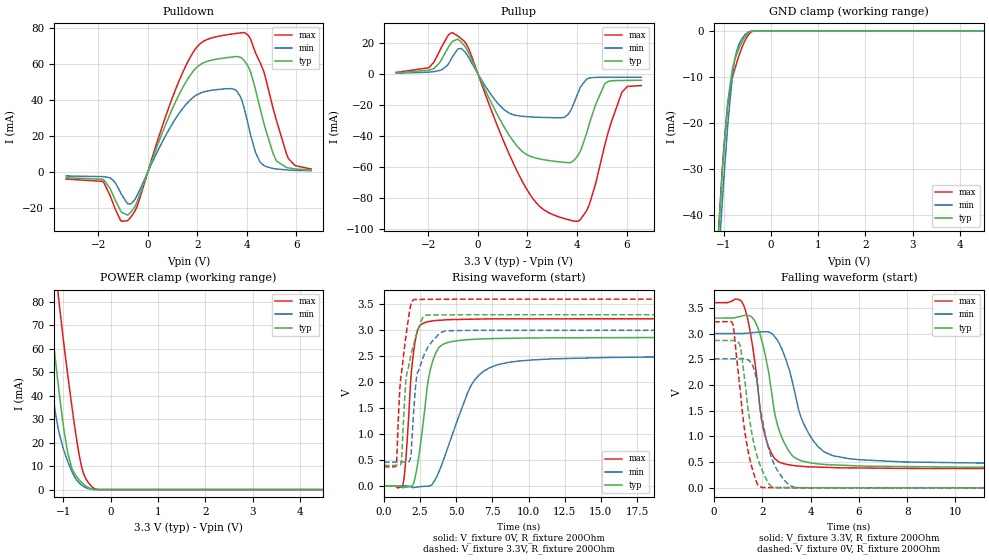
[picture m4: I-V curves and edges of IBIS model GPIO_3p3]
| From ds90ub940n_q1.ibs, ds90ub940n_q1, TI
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|   Model
[Model]   GPIO_3p3
Model_type   I/O
Polarity   Non-Inverting
Enable   Active-Low
Vinl = 0.8
Vinh = 2.0
Vmeas = 1.65
Vref = 0
Cref = 1pF
Rref = 100000
|   typ   min   max
C_comp   1.5999pF   1.5084pF   1.9148pF
[Voltage Range]   3.3   3   3.6
[Temperature Range]   27   105   -40
[Pullup Reference]   3.3   3   3.6
[Pulldown Reference]   -0   0   0
[Power Clamp Reference]   3.3   3   3.6
[GND Clamp Reference]   0   0   0
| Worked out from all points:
|   slope of the pulldown table from 0 to 0.495 V, typ, clamps not added: 26.6 ohm
|   slope of the pullup table from 0 to 0.495 V, typ, clamps not added: 29 ohm
|   GND clamp passes 1 mA (typ) near -0.52 V on its own axis
|   POWER clamp passes 1 mA (typ) near -0.48 V on its own axis
|   falling waveform, V_fixture 3.3V, R_fixture 200Ohm: 20-80 % time 759ps typ, 1.06ns min, 587ps max; typ from 3.3 V to 0.396 V
|   rising waveform, V_fixture 0V, R_fixture 200Ohm: 20-80 % time 842ps typ, 2.07ns min, 504ps max; typ from 0 V to 2.86 V
|   rising waveform, V_fixture 3.3V, R_fixture 200Ohm: 20-80 % time 741ps typ, 779ps min, 598ps max; typ from 0.395 V to 3.3 V
|   falling waveform, V_fixture 0V, R_fixture 200Ohm: 20-80 % time 590ps typ, 660ps min, 516ps max; typ from 2.87 V to 0 V
[Pulldown]
|   Voltage   I(typ)   I(min)   I(max)
-3.3V     -3.164mA   -2.173mA   -3.905mA
-1.835V   -3.993mA   -2.542mA   -5.143mA
-1.112V   -21.25mA   -11.09mA   -26.52mA
-815.1mV  -23.91mA   -17.65mA   -27.01mA
-429mV    -16.44mA   -12.96mA   -18.93mA
1.818V    55.76mA    41.37mA    66.26mA
3.482V    64.03mA    46.04mA    76.84mA
3.877V    62.19mA    36.29mA    77.51mA
4.531V    35.47mA    5.597mA    60.97mA
5.184V    6.455mA    1.721mA    29.19mA
5.679V    2.299mA    1.122mA    7.433mA
6.6V      1.091mA    735.9uA    1.663mA
[GND Clamp]
|   Voltage   I(typ)   I(min)   I(max)
-3.3V     -490.9mA   -454.2mA   -525.1mA
-1.122V   -47.07mA   -52.59mA   -46.26mA
-1.033V   -32.05mA   -38.23mA   -31.12mA
-993.3mV  -26.03mA   -32.18mA   -25.39mA
-914.1mV  -15.95mA   -21mA      -16.38mA
-815.1mV  -8.436mA   -9.999mA   -10.35mA
-755.7mV  -6.108mA   -5.891mA   -8.109mA
-686.4mV  -4.119mA   -3.295mA   -5.787mA
-577.5mV  -1.834mA   -1.244mA   -2.814mA
-458.7mV  -332.6uA   -204.8uA   -676.2uA
-260.7mV  -1.284uA   -1.62uA    -2.04uA
6.6V      0A         0A         0A
[Pullup]
|   Voltage   I(typ)   I(min)   I(max)
-3.3V     727.6uA    454.7uA    986.5uA
-1.993V   2.271mA    1.124mA    3.904mA
-1.468V   9.315mA    2.642mA    17.31mA
-676.5mV  20.61mA    16.42mA    22.71mA
768.9mV   -25.77mA   -18.3mA    -32.8mA
1.68V     -48.24mA   -27.07mA   -65.82mA
2.511V    -54.85mA   -27.98mA   -85.64mA
3.897V    -55.4mA    -18mA      -94.88mA
4.501V    -32.01mA   -2.633mA   -84.1mA
5.115V    -6.534mA   -2.196mA   -46.4mA
5.818V    -4.217mA   -2.156mA   -11.71mA
6.6V      -4.115mA   -2.126mA   -7.516mA
[POWER Clamp]
|   Voltage   I(typ)   I(min)   I(max)
-3.3V     488.4mA    415.5mA    566.2mA
-1.676V   153.8mA    114.9mA    202.9mA
-1.409V   100.9mA    68.98mA    144.9mA
-1.35V    89.41mA    59.34mA    132.2mA
-1.231V   66.97mA    41.31mA    107.5mA
-1.102V   43.92mA    25.52mA    82.16mA
-973.5mV  23.72mA    15.84mA    59.7mA
-815.1mV  8.895mA    7.566mA    34.94mA
-636.9mV  3.54mA     2.322mA    11.95mA
-508.2mV  1.311mA    677.8uA    4.14mA
-260.7mV  6.871uA    4.277uA    41.53uA
6.6V      0A         0A         0A
[Ramp]
R_load = 200
|   typ   min   max
dV/dt_r   1.71827/8.41806e-10   1.50408/2.06636e-09   1.93592/5.02199e-10
dV/dt_f   1.74251/7.59472e-10   1.52289/1.05507e-09   1.93753/5.8591e-10
[Falling Waveform]
V_fixture = 3.3V
V_fixture_min = 3V
V_fixture_max = 3.6V
R_fixture = 200Ohm
C_fixture = 0F
|   Time   V(typ)   V(min)   V(max)
0s        3.3V       3V         3.6V
1.161ns   3.341V     3.001V     3.609V
1.693ns   3.239V     3.021V     2.43V
1.959ns   2.893V     3.032V     1.352V
2.26ns    2.25V      3.031V     798.1mV
2.611ns   1.252V     2.881V     531.3mV
3.175ns   667.5mV    2.191V     441.9mV
4.176ns   473.8mV    875.1mV    406mV
5.811ns   430.4mV    556.1mV    387.3mV
40ns      395.8mV    461.8mV    370.8mV
[Rising Waveform]
V_fixture = 0V
V_fixture_min = 0V
V_fixture_max = 0V
R_fixture = 200Ohm
C_fixture = 0F
|   Time   V(typ)   V(min)   V(max)
0s        -6.538uV   984.3nV    3.936uV
1.291ns   -31.74mV   17.28uV    2.32mV
1.505ns   -25.18mV   19.97uV    480.4mV
1.863ns   -6.233mV   -16.06mV   2.073V
2.085ns   86.31mV    -29.62mV   2.651V
2.983ns   1.882V     -4.527mV   3.161V
4.041ns   2.725V     442.5mV    3.197V
6.047ns   2.823V     1.949V     3.213V
7.86ns    2.842V     2.337V     3.22V
40ns      2.864V     2.507V     3.227V
[Rising Waveform]
V_fixture = 3.3V
V_fixture_min = 3V
V_fixture_max = 3.6V
R_fixture = 200Ohm
C_fixture = 0F
|   Time   V(typ)   V(min)   V(max)
0s        395.4mV    460.8mV    370.5mV
856.2ps   394.2mV    460.6mV    416.7mV
1.182ns   433mV      460.6mV    2.118V
1.548ns   2.109V     460.5mV    2.943V
1.857ns   2.508V     578.2mV    3.49V
2.085ns   2.76V      1.548V     3.591V
2.272ns   2.928V     2.129V     3.594V
2.811ns   3.275V     2.549V     3.595V
4.327ns   3.296V     2.991V     3.598V
40ns      3.3V       3V         3.6V
[Falling Waveform]
|Gnd
V_fixture = 0V
V_fixture_min = 0V
V_fixture_max = 0V
R_fixture = 200Ohm
C_fixture = 0F
|   Time   V(typ)   V(min)   V(max)
0s        2.865V     2.507V     3.227V
778.2ps   2.865V     2.507V     3.182V
1.065ns   2.779V     2.508V     1.972V
1.291ns   2.016V     2.504V     1.041V
1.599ns   977.6mV    2.382V     342.6mV
1.983ns   351.9mV    1.371V     7.952mV
2.272ns   80.19mV    743mV      5.622mV
2.605ns   6.005mV    352.9mV    4.524mV
3.487ns   3.202mV    5.159mV    1.615mV
40ns      -4.17uV    984.3nV    5.812uV
